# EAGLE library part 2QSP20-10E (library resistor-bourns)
BOURNS RESISTOR NETWORK
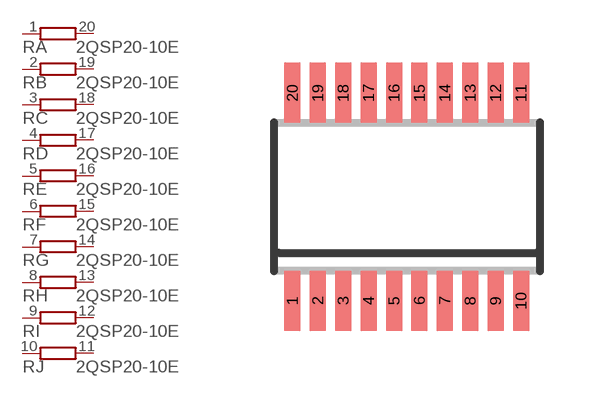
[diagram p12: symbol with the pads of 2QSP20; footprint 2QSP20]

Designator prefix R; gates A=R1NV B=R1NV C=R1NV D=R1NV E=R1NV F=R1NV G=R1NV H=R1NV I=R1NV J=R1NV

## 2QSP20-10E (OC_FARNELL: unknown; OC_NEWARK: unknown)  [2QSP20]
1  A:1  pas
2  B:1  pas
3  C:1  pas
4  D:1  pas
5  E:1  pas
6  F:1  pas
7  G:1  pas
8  H:1  pas
9  I:1  pas
10  J:1  pas
11  J:2  pas
12  I:2  pas
13  H:2  pas
14  G:2  pas
15  F:2  pas
16  E:2  pas
17  D:2  pas
18  C:2  pas
19  B:2  pas
20  A:2  pas

## Footprint 2QSP20 (pad centres in mm)
BOURNS RESISTOR NETWORK
smd 0.4 x 1.5: 1 -2.223,-2.6; 2 -1.588,-2.6; 3 -0.953,-2.6; 4 -0.318,-2.6; 5 0.318,-2.6; 6 0.953,-2.6; 7 1.588,-2.6; 8 2.223,-2.6; 9 2.858,-2.6; 10 3.493,-2.6; 11 3.493,2.6; 12 2.858,2.6; 13 2.223,2.6; 14 1.588,2.6; 15 0.953,2.6; 16 0.318,2.6; 17 -0.318,2.6; 18 -0.953,2.6; 19 -1.588,2.6; 20 -2.223,2.6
